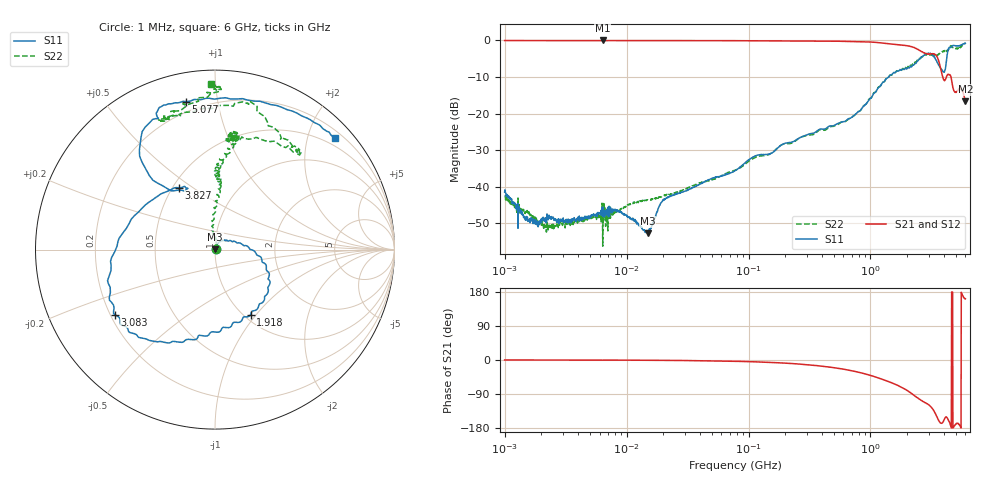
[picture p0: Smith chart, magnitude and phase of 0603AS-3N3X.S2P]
!s-Parameter Generated by FASTRON Sdn. Bhd.
!FASTRON P/N : 0603AS-3N3X
!Keysight Technologies: E5071C_MY46733604_B.14.02
!Date: Tue Nov 21 14:58:44 2023
!Version  :Rev01  Tue Nov 21 14:58:44 2023
!Data & Calibration Information:
!Freq  S11:SOLT2(ON)  S21:SOLT2(ON)  S12:SOLT2(ON)  S22:SOLT2(ON)
!PortZ  Port1:50+j0  Port2:50+j0
!When reading reference impedance value at option line is always used.
! Remarks : This data is being provided solely for informational purposes.
# Hz S dB R 50
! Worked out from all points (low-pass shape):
!   1601 points, 1 MHz to 6 GHz, reference 50 ohm
!   highest |S21| = -0.01 dB at 6.378 MHz (marker M1); lowest = -16.7 dB at 6 GHz (marker M2)
!   |S21| within 3 dB of the highest: start of sweep to 2.604 GHz
!   lowest |S11| = -52.8 dB at 14.93 MHz (marker M3), VSWR 1.00, Z = 50.2 + j0.157 ohm
!   |S11| at or under -10 dB: start of sweep to 1.408 GHz
!   |S22| runs from -56.2 to -0.7 dB; largest |S21 - S12| = 0.011
!   S11 on the Smith chart (normalised r, x): 1 MHz: 1.02, +0.01; 1.918 GHz: 1.07, -0.94; 3.083 GHz: 0.22, -0.28; 3.827 GHz: 0.54, +0.44; 5.077 GHz: 0.15, +0.81; 6 GHz: 0.34, +2.51
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1000000  -41.40 18.6  -0.03 0.1  -0.05 0.2  -42.45 24.2
1819981  -49.20 12.3  -0.04 -0.0  -0.05 0.0  -48.56 2.0
2178434  -49.19 36.6  -0.05 -0.1  -0.05 -0.0  -50.93 43.0
4277066  -48.94 31.3  -0.05 -0.2  -0.05 -0.2  -49.35 39.9
6378092  -48.11 48.9  -0.01 -0.3  -0.06 -0.4  -56.24 30.6
8700030  -46.65 38.2  -0.04 -0.4  -0.05 -0.4  -46.42 42.4
1.493236e7  -52.76 43.0  -0.04 -0.7  -0.05 -0.7  -43.56 33.5
1.823719e7  -45.85 46.5  -0.05 -0.9  -0.06 -0.8  -42.89 47.3
2.231736e7  -42.76 48.9  -0.05 -1.1  -0.06 -1.0  -42.13 57.3
7.757876e7  -35.64 61.2  -0.07 -3.4  -0.08 -3.4  -35.50 62.2
3.307917e8  -25.40 55.7  -0.16 -13.5  -0.16 -13.5  -25.79 83.5
7.165695e8  -20.72 31.9  -0.28 -28.9  -0.28 -28.9  -20.80 97.7
1.414819e9  -9.90 -22.6  -0.91 -57.5  -0.92 -57.5  -9.96 85.0
1.918046e9  -7.69 -61.2  -1.40 -77.0  -1.41 -77.0  -7.56 86.6
2.599543e9  -4.68 -117.0  -2.99 -106.5  -2.99 -106.3  -4.58 79.8
3.083002e9  -3.53 -147.0  -3.76 -121.5  -3.72 -121.5  -3.65 79.5
3.482718e9  -5.62 170.2  -4.29 -147.9  -4.27 -148.2  -3.98 81.4
3.826954e9  -7.99 120.2  -8.70 -167.5  -8.70 -167.8  -3.28 57.2
4.19144e9  -5.70 131.8  -9.95 -150.2  -9.97 -150.5  -2.96 53.2
4.517068e9  -1.97 113.3  -9.54 -170.8  -9.57 -171.0  -1.60 73.6
5.076665e9  -1.51 101.1  -14.01 -167.8  -14.06 -167.8  -2.27 109.6
6e9  -0.80 42.9  -16.66 161.3  -16.64 161.4  -0.71 91.2
